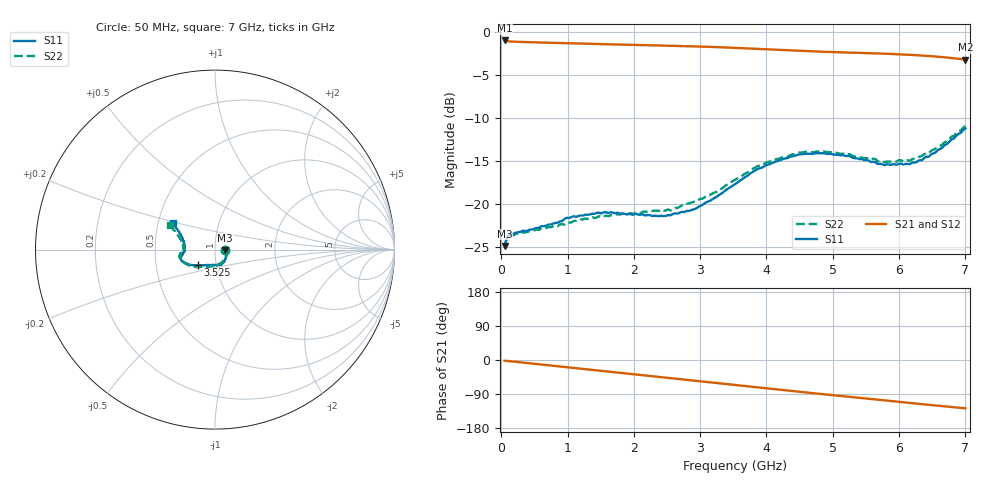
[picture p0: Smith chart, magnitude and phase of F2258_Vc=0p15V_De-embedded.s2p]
! Integrated Device Technology
! Corporate Headquarters
! 6024 Silver Creek Valley Road
! San Jose, CA 95138  USA
! Phone:  1-408-284-8200
! Toll Free:  1-800-223-1366
! Webpage:  http://www.idt.com/
! Timing and RF Division
! 515 Groton Road, Suite 102
! Westford, MA 01886-6024
! Device:  F2258
! Description: Voltage Variable RF Attenuator
! Frequency:  50.0 -  6000.00 MHz
! Package:  3x3 mm Thin QFN Plastic Package: 16 pin
! Ports:  2 RF, 2 DC
!  Pin  1  = NC
!  Pin  2  = NC
!  Pin  3  = RF2  = Port 2
!  Pin  4  = GND
!  Pin  5  = Vdd
!  Pin  6  = NC
!  Pin  7  = VCTRL
!  Pin  8  = NC
!  Pin  9  = GND
!  Pin 10  = RF1  = Port 1
!  Pin 11  = NC
!  Pin 12  = NC
!  Pin 13  = NC
!  Pin 14  = NC
!  Pin 15  = NC
!  Pin 16  = NC
! Vcntrl:  0.150 Volts
! Vdd:  +3.300 Volts
! Current:  1.074 mA
! Data:  The device was measured on a the F2258 evaluation board which has
!  individual transmission lines to the RF pins.  Data was collected
!  using a calibrated network analyzer.  The evaluation board was
!  de-embedded using a TRL calibration technique.
!  The reference plane is the edge of the package pin.
! Misc:  SN 10
!  Action Tracker AT0285
! Date Measured:  2014-12-10
! Date:  2016-01-13  MJV
! Note:
!  Integrated Device Technology supplies this data as a sample of measured
!  data at the package pin for this product.  Your particular data for this
!  product may vary.
!  Data was taken at 25 degrees C.
!  Integrated Device Technology reserves the right to change this data at anytime.
!Freq_(GHz)  S11M_(dB)  S11P_(deg)  S21M_(dB)  S21P_(deg)  S12M_(dB)  S12P_(deg)  S22M_(dB)  S22P_(deg)
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# GHz S dB R 50
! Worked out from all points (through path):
!   201 points, 50 MHz to 7 GHz, reference 50 ohm
!   highest |S21| = -0.96 dB at 50 MHz (marker M1); lowest = -3.2 dB at 7 GHz (marker M2)
!   group delay of S21, straight-line fit = 50.5 ps
!   lowest |S11| = -24.9 dB at 50 MHz (marker M3), VSWR 1.12, Z = 56 - j0.391 ohm
!   |S11| at or under -10 dB: start of sweep to end of sweep
!   |S22| runs from -24.9 to -10.9 dB; largest |S21 - S12| = 0.00033
!   S11 on the Smith chart (normalised r, x): 50 MHz: 1.12, -0.01; 3.525 GHz: 0.81, -0.14; 7 GHz: 0.60, +0.19
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0.05  -24.87 -3.5  -0.96 -1.9  -0.96 -1.9  -24.91 -3.0
0.08475  -23.89 -6.0  -1.03 -2.4  -1.03 -2.4  -23.97 -5.4
0.15425  -23.41 -9.3  -1.08 -3.6  -1.08 -3.6  -23.59 -9.4
0.71025  -22.39 -37.2  -1.22 -14.1  -1.22 -14.1  -22.69 -38.6
0.98825  -21.60 -51.0  -1.27 -19.3  -1.27 -19.3  -22.17 -54.7
1.2315  -21.35 -59.3  -1.32 -23.8  -1.32 -23.8  -21.80 -63.7
1.6485  -20.94 -71.0  -1.41 -31.4  -1.41 -31.4  -21.32 -76.8
2.37825  -21.41 -92.5  -1.54 -44.8  -1.54 -44.8  -20.78 -94.3
2.552  -21.31 -98.5  -1.57 -48.0  -1.57 -48.0  -20.74 -99.6
2.93425  -20.53 -115.1  -1.65 -55.1  -1.65 -55.1  -19.73 -112.9
3.525  -17.70 -137.8  -1.82 -66.2  -1.82 -66.2  -17.21 -135.6
4.0115  -15.43 -151.4  -2.00 -75.2  -2.00 -75.2  -15.12 -151.0
4.46325  -14.28 -159.8  -2.16 -83.4  -2.16 -83.4  -14.07 -162.1
4.7065  -14.15 -163.1  -2.23 -87.7  -2.23 -87.7  -13.96 -166.3
5.15825  -14.31 -168.5  -2.35 -95.6  -2.35 -95.6  -14.14 -173.2
5.64475  -15.15 -176.7  -2.47 -104.0  -2.47 -104.0  -14.77 -179.4
5.6795  -15.35 -176.8  -2.47 -104.6  -2.47 -104.6  -15.03 -179.7
5.85325  -15.41 179.0  -2.52 -107.8  -2.52 -107.8  -15.06 175.7
6.166  -15.34 171.2  -2.63 -113.4  -2.63 -113.4  -14.97 169.8
6.33975  -14.93 164.9  -2.71 -116.5  -2.71 -116.5  -14.43 165.4
6.722  -13.01 153.3  -2.95 -123.1  -2.94 -123.1  -12.71 156.4
7  -11.19 147.9  -3.19 -127.4  -3.19 -127.4  -10.92 151.5
